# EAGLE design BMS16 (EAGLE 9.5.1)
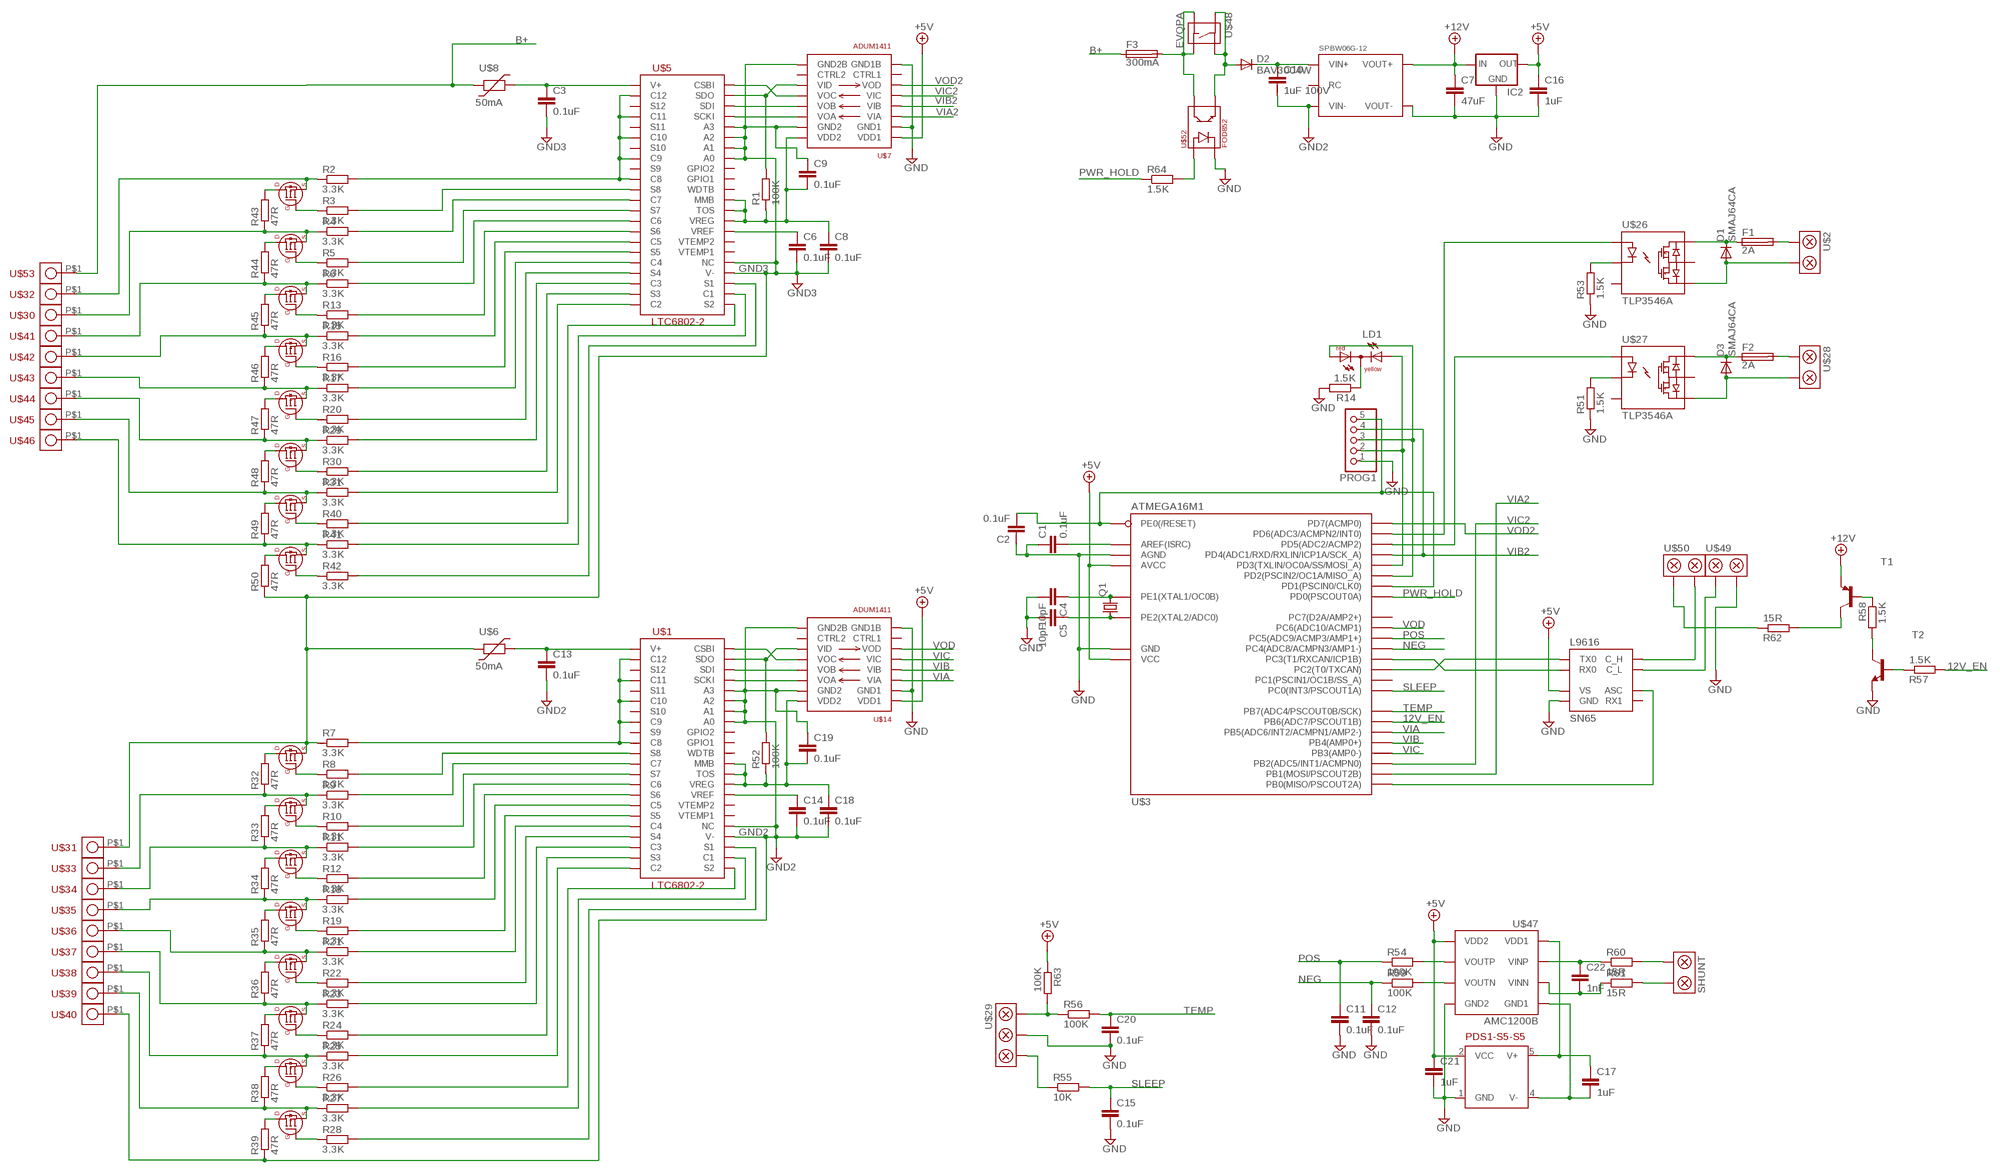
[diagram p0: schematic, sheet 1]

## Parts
C1  0.1uF  C-EUC1206  [C1206]
C2  0.1uF  C-EUC1206  [C1206]
C3  0.1uF  C-EUC1206  [C1206]
C4  10pF  C-EUC0805  [C0805]
C5  10pF  C-EUC0805  [C0805]
C6  0.1uF  C-EUC1206  [C1206]
C7  47uF  C-EUC1206  [C1206]
C8  0.1uF  C-EUC1206  [C1206]
C9  0.1uF  C-EUC1206  [C1206]
C10  1uF 100V  C-EUC1206  [C1206]
C11  0.1uF  C-EUC1206  [C1206]
C12  0.1uF  C-EUC1206  [C1206]
C13  0.1uF  C-EUC1206  [C1206]
C14  0.1uF  C-EUC1206  [C1206]
C15  0.1uF  C-EUC1206  [C1206]
C16  1uF  C-EUC1206  [C1206]
C17  1uF  C-EUC1206  [C1206]
C18  0.1uF  C-EUC1206  [C1206]
C19  0.1uF  C-EUC1206  [C1206]
C20  0.1uF  C-EUC1206  [C1206]
C21  1uF  C-EUC1206  [C1206]
C22  1nF  C-EUC1206  [C1206]
D1  SMAJ64CA  DIODE-DO214AC  [DO214AC]
D2  BAV3004W  DIODE-SOD123  [SOD123]
D3  SMAJ64CA  DIODE-DO214AC  [DO214AC]
F1  2A  TE5  [TE5]
F2  2A  TE5  [TE5]
F3  300mA  TE5  [TE5]
IC2  78LXXSOT89  [SOT89R]
LD1  DUOLED-RY-C  [DUOLED-C-5MM]
PDS1-S5-S5  PDS2  [PDS2]
PROG1  PINHD-1X5  [1X05]
Q1  CRYSTALCTS406  [CTS406]
R1  100K  R-EU_R1206  [R1206]
R2  3.3K  R-EU_R1206  [R1206]
R3  3.3K  R-EU_R1206  [R1206]
R4  3.3K  R-EU_R1206  [R1206]
R5  3.3K  R-EU_R1206  [R1206]
R6  3.3K  R-EU_R1206  [R1206]
R7  3.3K  R-EU_R1206  [R1206]
R8  3.3K  R-EU_R1206  [R1206]
R9  3.3K  R-EU_R1206  [R1206]
R10  3.3K  R-EU_R1206  [R1206]
R11  3.3K  R-EU_R1206  [R1206]
R12  3.3K  R-EU_R1206  [R1206]
R13  3.3K  R-EU_R1206  [R1206]
R14  1.5K  R-EU_R1206  [R1206]
R15  3.3K  R-EU_R1206  [R1206]
R16  3.3K  R-EU_R1206  [R1206]
R17  3.3K  R-EU_R1206  [R1206]
R18  3.3K  R-EU_R1206  [R1206]
R19  3.3K  R-EU_R1206  [R1206]
R20  3.3K  R-EU_R1206  [R1206]
R21  3.3K  R-EU_R1206  [R1206]
R22  3.3K  R-EU_R1206  [R1206]
R23  3.3K  R-EU_R1206  [R1206]
R24  3.3K  R-EU_R1206  [R1206]
R25  3.3K  R-EU_R1206  [R1206]
R26  3.3K  R-EU_R1206  [R1206]
R27  3.3K  R-EU_R1206  [R1206]
R28  3.3K  R-EU_R1206  [R1206]
R29  3.3K  R-EU_R1206  [R1206]
R30  3.3K  R-EU_R1206  [R1206]
R31  3.3K  R-EU_R1206  [R1206]
R32  47R  R-EU_R2512  [R2512]
R33  47R  R-EU_R2512  [R2512]
R34  47R  R-EU_R2512  [R2512]
R35  47R  R-EU_R2512  [R2512]
R36  47R  R-EU_R2512  [R2512]
R37  47R  R-EU_R2512  [R2512]
R38  47R  R-EU_R2512  [R2512]
R39  47R  R-EU_R2512  [R2512]
R40  3.3K  R-EU_R1206  [R1206]
R41  3.3K  R-EU_R1206  [R1206]
R42  3.3K  R-EU_R1206  [R1206]
R43  47R  R-EU_R2512  [R2512]
R44  47R  R-EU_R2512  [R2512]
R45  47R  R-EU_R2512  [R2512]
R46  47R  R-EU_R2512  [R2512]
R47  47R  R-EU_R2512  [R2512]
R48  47R  R-EU_R2512  [R2512]
R49  47R  R-EU_R2512  [R2512]
R50  47R  R-EU_R2512  [R2512]
R51  1.5K  R-EU_R1206  [R1206]
R52  100K  R-EU_R1206  [R1206]
R53  1.5K  R-EU_R1206  [R1206]
R54  100K  R-EU_R1206  [R1206]
R55  10K  R-EU_R1206  [R1206]
R56  100K  R-EU_R1206  [R1206]
R57  1.5K  R-EU_R1206  [R1206]
R58  1.5K  R-EU_R1206  [R1206]
R59  100K  R-EU_R1206  [R1206]
R60  15R  R-EU_R1206  [R1206]
R61  15R  R-EU_R1206  [R1206]
R62  15R  R-EU_R1206  [R1206]
R63  100K  R-EU_R1206  [R1206]
R64  1.5K  R-EU_R1206  [R1206]
SHUNT  SCREWTERM_2WAY5MM  [SCREWTERM_5MM_2WAY]
SN65  L9616  [SOIC8]
SPBW06G-12  SPBW06  [SPBW06]
T1  MMBT540LT1-PNP-SOT23-BEC  [SOT23-BEC]
T2  MMBT4401LT1-NPN-SOT23-BEC  [SOT23-BEC]
U$1  LTC6802-2  [SSOP-44]
U$2  SCREWTERM_2WAY5MM  [SCREWTERM_5MM_2WAY]
U$3  ATMEGA16M1  [TQFP32]
U$5  LTC6802-2  [SSOP-44]
U$6  50mA  1206_POLYSWITCH  [1206]
U$7  ADUM1411  [SOIC16W]
U$8  50mA  1206_POLYSWITCH  [1206]
U$9  SI2351DS  [SOT23]
U$10  SI2351DS  [SOT23]
U$11  SI2351DS  [SOT23]
U$12  SI2351DS  [SOT23]
U$13  SI2351DS  [SOT23]
U$14  ADUM1411  [SOIC16W]
U$15  SI2351DS  [SOT23]
U$16  SI2351DS  [SOT23]
U$17  SI2351DS  [SOT23]
U$18  SI2351DS  [SOT23]
U$19  SI2351DS  [SOT23]
U$20  SI2351DS  [SOT23]
U$21  SI2351DS  [SOT23]
U$22  SI2351DS  [SOT23]
U$23  SI2351DS  [SOT23]
U$24  SI2351DS  [SOT23]
U$25  SI2351DS  [SOT23]
U$26  TLP3546A  AQV252GA  [SMD6]
U$27  TLP3546A  AQV252GA  [SMD6]
U$28  SCREWTERM_2WAY5MM  [SCREWTERM_5MM_2WAY]
U$29  SCREWTERM_3WAY5MM  [SCREWTERM_5MM_3WAY]
U$30  PHOENIX_508_SCREW_PLUG_1  [PHOENIX_508_SCREW_PLUG_1]
U$31  PHOENIX_508_SCREW_PLUG_1  [PHOENIX_508_SCREW_PLUG_1]
U$32  PHOENIX_508_SCREW_PLUG_1  [PHOENIX_508_SCREW_PLUG_1]
U$33  PHOENIX_508_SCREW_PLUG_1  [PHOENIX_508_SCREW_PLUG_1]
U$34  PHOENIX_508_SCREW_PLUG_1  [PHOENIX_508_SCREW_PLUG_1]
U$35  PHOENIX_508_SCREW_PLUG_1  [PHOENIX_508_SCREW_PLUG_1]
U$36  PHOENIX_508_SCREW_PLUG_1  [PHOENIX_508_SCREW_PLUG_1]
U$37  PHOENIX_508_SCREW_PLUG_1  [PHOENIX_508_SCREW_PLUG_1]
U$38  PHOENIX_508_SCREW_PLUG_1  [PHOENIX_508_SCREW_PLUG_1]
U$39  PHOENIX_508_SCREW_PLUG_1  [PHOENIX_508_SCREW_PLUG_1]
U$40  PHOENIX_508_SCREW_PLUG_1  [PHOENIX_508_SCREW_PLUG_1]
U$41  PHOENIX_508_SCREW_PLUG_1  [PHOENIX_508_SCREW_PLUG_1]
U$42  PHOENIX_508_SCREW_PLUG_1  [PHOENIX_508_SCREW_PLUG_1]
U$43  PHOENIX_508_SCREW_PLUG_1  [PHOENIX_508_SCREW_PLUG_1]
U$44  PHOENIX_508_SCREW_PLUG_1  [PHOENIX_508_SCREW_PLUG_1]
U$45  PHOENIX_508_SCREW_PLUG_1  [PHOENIX_508_SCREW_PLUG_1]
U$46  PHOENIX_508_SCREW_PLUG_1  [PHOENIX_508_SCREW_PLUG_1]
U$47  AMC1200B  AMC1200  [SOIC8W]
U$48  EVQPA  [EVQPA]
U$49  SCREWTERM_2WAY5MM  [SCREWTERM_5MM_2WAY]
U$50  SCREWTERM_2WAY5MM  [SCREWTERM_5MM_2WAY]
U$52  FOD852  [SMD4]
U$53  PHOENIX_508_SCREW_PLUG_1  [PHOENIX_508_SCREW_PLUG_1]

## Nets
12V_EN: R57.2 U$3.27(PB6(ADC7/PSCOUT1B))
+5V: C16.1 C21.1 IC2.2(OUT) PDS1-S5-S5.2(VCC) R63.1 SN65.P$3(VS) U$3.4(VCC) U$3.19(AVCC) U$7.1(VDD1) U$14.1(VDD1) U$47.8(VDD2)
+12V: C7.1 IC2.1(IN) SPBW06G-12.6(VOUT+) T1.E
B+: F3.1 U$8.P$1 U$53.P$1
FD: F3.2 U$48.A U$48.A2 U$52.P$4(COL)
FDS: C3.1 U$5.1(V+) U$8.P$2
FS: R2.1 U$18.P$2(S) U$32.P$1
GND: C1.1 C2.1 C4.2 C5.2 C7.2 C11.2 C12.2 C15.2 C16.2 C20.2 C21.2 IC2.4(GND) PDS1-S5-S5.1(GND) PROG1.1 R14.2 R51.1 R53.1 SN65.P$2(GND) SPBW06G-12.7(VOUT-) T2.E U$3.5(GND) U$3.20(AGND) U$7.2(GND1) U$7.8(GND1B) U$14.2(GND1) U$14.8(GND1B) U$29.P$2 U$47.5(GND2) U$49.P$1 U$52.P$2(CAT)
GND2: C10.2 C13.2 C14.2 C18.2 C19.1 R39.1 SPBW06G-12.1(VIN-) U$1.26(V-) U$1.27(NC) U$1.37(A0) U$1.38(A1) U$1.39(A2) U$1.40(A3) U$14.9(GND2B) U$14.15(GND2) U$40.P$1
GND3: C3.2 C6.2 C8.2 C9.1 R7.1 R50.1 U$5.26(V-) U$5.27(NC) U$5.37(A0) U$5.38(A1) U$5.39(A2) U$5.40(A3) U$6.P$1 U$7.9(GND2B) U$7.15(GND2) U$9.P$2(S) U$31.P$1
N$1: D1.C F1.1 U$26.6
N$2: R7.2 U$1.2(C12) U$1.4(C11) U$1.6(C10) U$1.8(C9) U$1.10(C8)
N$3: C22.1 R60.1 U$47.2(VINP)
N$4: U$5.42(SDI) U$7.13(VOB)
N$5: U$5.41(SCKI) U$7.14(VOA)
N$6: R1.2 U$5.43(SDO) U$7.11(VID)
N$7: U$1.42(SDI) U$14.13(VOB)
N$8: U$5.44(CSBI) U$7.12(VOC)
N$9: C8.1 C9.2 R1.1 U$5.31(VREG) U$5.32(TOS) U$5.33(MMB) U$7.16(VDD2)
N$10: R26.2 U$1.23(S2)
N$11: U$1.41(SCKI) U$14.14(VOA)
N$12: R27.2 U$1.24(C1)
N$13: R28.2 U$1.25(S1)
N$14: C6.1 U$5.30(VREF)
N$15: R52.2 U$1.43(SDO) U$14.11(VID)
N$16: U$1.44(CSBI) U$14.12(VOC)
N$17: R40.2 U$5.23(S2)
N$18: R41.2 U$5.24(C1)
N$19: C2.2 PROG1.5 U$3.31(PE0(/RESET)) U$3.32(PD1(PSCIN0/CLK0))
N$20: F1.2 U$2.P$2
N$21: R42.2 U$5.25(S1)
N$22: R4.2 U$5.12(C7)
N$23: R9.2 U$1.12(C7)
N$24: R11.2 U$1.14(C6)
N$25: C18.1 C19.2 R52.1 U$1.31(VREG) U$1.32(TOS) U$1.33(MMB) U$14.16(VDD2)
N$26: R18.2 U$1.16(C5)
N$27: R21.2 U$1.18(C4)
N$28: R23.2 U$1.20(C3)
N$29: R25.2 U$1.22(C2)
N$30: R6.2 U$5.14(C6)
N$31: R15.2 U$5.16(C5)
N$32: LD1.AX(AY) PROG1.2 U$3.2(PD3(TXLIN/OC0A/SS/MOSI_A))
N$33: LD1.AR PROG1.3 U$3.1(PD2(PSCIN2/OC1A/MISO_A))
N$34: F2.2 U$28.P$2
N$35: C1.2 U$3.21(AREF(ISRC))
N$36: SN65.P$4(RX0) U$3.7(PC3(T1/RXCAN/ICP1B))
N$37: SN65.P$1(TX0) U$3.6(PC2(T0/TXCAN))
N$38: SN65.P$7(C_H) U$50.P$1
N$39: SN65.P$6(C_L) U$49.P$2
N$40: C22.2 R61.1 U$47.3(VINN)
N$41: R55.1 U$29.P$1
N$42: C10.1 D2.C SPBW06G-12.2(VIN+)
N$43: D2.A U$48.B U$48.B2 U$52.P$3(EM)
N$44: R62.1 U$50.P$2
N$45: LD1.C R14.1
N$46: R17.2 U$5.18(C4)
N$47: SN65.P$8(ASC) U$3.8(PB0(MISO/PSCOUT2A))
N$48: C4.1 Q1.3 U$3.10(PE1(XTAL1/OC0B))
N$49: C5.1 Q1.1 U$3.11(PE2(XTAL2/ADC0))
N$50: R29.2 U$5.20(C3)
N$51: R31.2 U$5.22(C2)
N$52: R54.2 U$47.7(VOUTP)
N$53: D1.A U$2.P$1 U$26.4
N$54: R3.1 U$18.P$1(G)
N$55: R5.1 U$19.P$1(G)
N$56: R13.1 U$20.P$1(G)
N$57: R8.1 U$9.P$1(G)
N$58: R10.1 U$10.P$1(G)
N$59: R12.1 U$11.P$1(G)
N$60: R28.1 U$17.P$1(G)
N$61: R19.1 U$12.P$1(G)
N$62: R22.1 U$13.P$1(G)
N$63: R24.1 U$15.P$1(G)
N$64: R26.1 U$16.P$1(G)
N$65: R27.1 R38.1 U$17.P$2(S) U$39.P$1
N$66: C14.1 U$1.30(VREF)
N$67: R42.1 U$25.P$1(G)
N$68: R16.1 U$21.P$1(G)
N$69: R25.1 R37.1 U$16.P$2(S) U$38.P$1
N$70: R23.1 R36.1 U$15.P$2(S) U$37.P$1
N$71: R38.2 U$16.P$3(D)
N$72: R39.2 U$17.P$3(D)
N$73: R37.2 U$15.P$3(D)
N$74: R21.1 R35.1 U$13.P$2(S) U$36.P$1
N$75: R36.2 U$13.P$3(D)
N$76: R18.1 R34.1 U$12.P$2(S) U$35.P$1
N$77: R35.2 U$12.P$3(D)
N$78: R11.1 R33.1 U$11.P$2(S) U$34.P$1
N$79: R9.1 R32.1 U$10.P$2(S) U$33.P$1
N$80: R33.2 U$10.P$3(D)
N$81: R34.2 U$11.P$3(D)
N$82: R32.2 U$9.P$3(D)
N$83: R24.2 U$1.21(S3)
N$84: R22.2 U$1.19(S4)
N$85: R20.1 U$22.P$1(G)
N$86: R30.1 U$23.P$1(G)
N$87: R40.1 U$24.P$1(G)
N$88: R41.1 R49.1 U$25.P$2(S) U$46.P$1
N$89: R8.2 U$1.11(S8)
N$90: R10.2 U$1.13(S7)
N$91: R12.2 U$1.15(S6)
N$92: R31.1 R48.1 U$24.P$2(S) U$45.P$1
N$93: R19.2 U$1.17(S5)
N$94: R29.1 R47.1 U$23.P$2(S) U$44.P$1
N$95: R49.2 U$24.P$3(D)
N$96: R50.2 U$25.P$3(D)
N$97: R48.2 U$23.P$3(D)
N$98: R17.1 R46.1 U$22.P$2(S) U$43.P$1
N$99: R47.2 U$22.P$3(D)
N$100: R15.1 R45.1 U$21.P$2(S) U$42.P$1
N$101: R46.2 U$21.P$3(D)
N$102: R6.1 R44.1 U$20.P$2(S) U$41.P$1
N$103: R4.1 R43.1 U$19.P$2(S) U$30.P$1
N$104: R44.2 U$19.P$3(D)
N$105: R45.2 U$20.P$3(D)
N$106: R43.2 U$18.P$3(D)
N$107: R3.2 U$5.11(S8)
N$108: R5.2 U$5.13(S7)
N$109: R13.2 U$5.15(S6)
N$110: R16.2 U$5.17(S5)
N$111: R20.2 U$5.19(S4)
N$112: R30.2 U$5.21(S3)
N$113: R2.2 U$5.2(C12) U$5.4(C11) U$5.6(C10) U$5.8(C9) U$5.10(C8)
N$114: R56.1 R63.2 U$29.P$3
N$115: D3.C F2.1 U$27.6
N$116: C17.1 PDS1-S5-S5.5(V+) U$47.1(VDD1)
N$117: D3.A U$27.4 U$28.P$1
N$118: U$3.14(PD6(ADC3/ACMPN2/INT0)) U$26.1
N$119: U$3.13(PD5(ADC2/ACMP2)) U$27.1
N$120: R53.2 U$26.2
N$121: R51.2 U$27.2
N$122: R57.1 T2.B
N$123: R58.2 T2.C
N$124: C17.2 PDS1-S5-S5.4(V-) U$47.4(GND1)
N$125: R58.1 T1.B
N$126: R62.2 T1.C
N$127: R59.2 U$47.6(VOUTN)
N$128: R64.2 U$52.P$1(AN)
N$129: R61.2 SHUNT.P$2
N$130: R60.2 SHUNT.P$1
NEG: C12.1 R59.1 U$3.17(PC4(ADC8/ACMPN3/AMP1-))
POS: C11.1 R54.1 U$3.18(PC5(ADC9/ACMP3/AMP1+))
PWR_HOLD: R64.1 U$3.29(PD0(PSCOUT0A))
SLEEP: C15.1 R55.2 U$3.30(PC0(INT3/PSCOUT1A))
TEMP: C20.1 R56.2 U$3.28(PB7(ADC4/PSCOUT0B/SCK))
V+: C13.1 U$1.1(V+) U$6.P$2
VIA: U$3.26(PB5(ADC6/INT2/ACMPN1/AMP2-)) U$14.3(VIA)
VIA2: U$3.9(PB1(MOSI/PSCOUT2B)) U$7.3(VIA)
VIB: U$3.24(PB4(AMP0+)) U$14.4(VIB)
VIB2: PROG1.4 U$3.12(PD4(ADC1/RXD/RXLIN/ICP1A/SCK_A)) U$7.4(VIB)
VIC: U$3.23(PB3(AMP0-)) U$14.5(VIC)
VIC2: U$3.16(PB2(ADC5/INT1/ACMPN0)) U$7.5(VIC)
VOD: U$3.22(PC6(ADC10/ACMP1)) U$14.6(VOD)
VOD2: U$3.15(PD7(ACMP0)) U$7.6(VOD)
Unconnected: SN65.P$5(RX1) SPBW06G-12.3(RC) U$1.3(S12) U$1.5(S11) U$1.7(S10) U$1.9(S9) U$1.28(VTEMP1) U$1.29(VTEMP2) U$1.34(WDTB) U$1.35(GPIO1) U$1.36(GPIO2) U$3.3(PC1(PSCIN1/OC1B/SS_A)) U$3.25(PC7(D2A/AMP2+)) U$5.3(S12) U$5.5(S11) U$5.7(S10) U$5.9(S9) U$5.28(VTEMP1) U$5.29(VTEMP2) U$5.34(WDTB) U$5.35(GPIO1) U$5.36(GPIO2) U$7.7(CTRL1) U$7.10(CTRL2) U$14.7(CTRL1) U$14.10(CTRL2) U$26.3 U$26.5 U$27.3 U$27.5

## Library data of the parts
C1-C22 = resistor:C-EU: CAPACITOR, European symbol
D1-D3 = diode:DIODE-: DIODE
F1-F3 = fuse:TE5: FUSE
IC2 = v-reg:78LXX: VOLTAGE REGULATOR
LD1 = led:DUOLED-RY-C: DUO LED 2 colors (red/yellow), 5 mm, round, common Cathode www.ligitek.com or other producers.
PDS1-S5-S5 = Ians parts:PDS2
PROG1 = pinhead:PINHD-1X5: PIN HEADER
Q1 = crystal:CRYSTAL: CRYSTAL
R1-R64 = resistor:R-EU_: RESISTOR, European symbol
SHUNT U$2 U$28 U$49 U$50 = Ians parts:SCREWTERM_2WAY
SN65 = Ians parts:L9616
SPBW06G-12 = Ians parts:SPBW06
T1 = transistor:*-PNP-: PNP Transistror
T2 = transistor:*-NPN-: NPN Transistror BF959 corrected 2008.03.06
U$1 U$5 = Ians parts:LTC6802-2
U$3 = Ians parts:ATMEGA16M1
U$6 U$8 = Ians parts:1206_POLYSWITCH
U$7 U$14 = Ians parts:ADUM1411
U$9-U$13 U$15-U$25 = Ians parts:SI2351DS
U$26 U$27 = Ians parts:AQV252GA
U$29 = Ians parts:SCREWTERM_3WAY
U$30-U$46 U$53 = Ians parts:PHOENIX_508_SCREW_PLUG_1
U$47 = Ians parts:AMC1200
U$48 = Ians parts:EVQPA
U$52 = Ians parts:FOD852

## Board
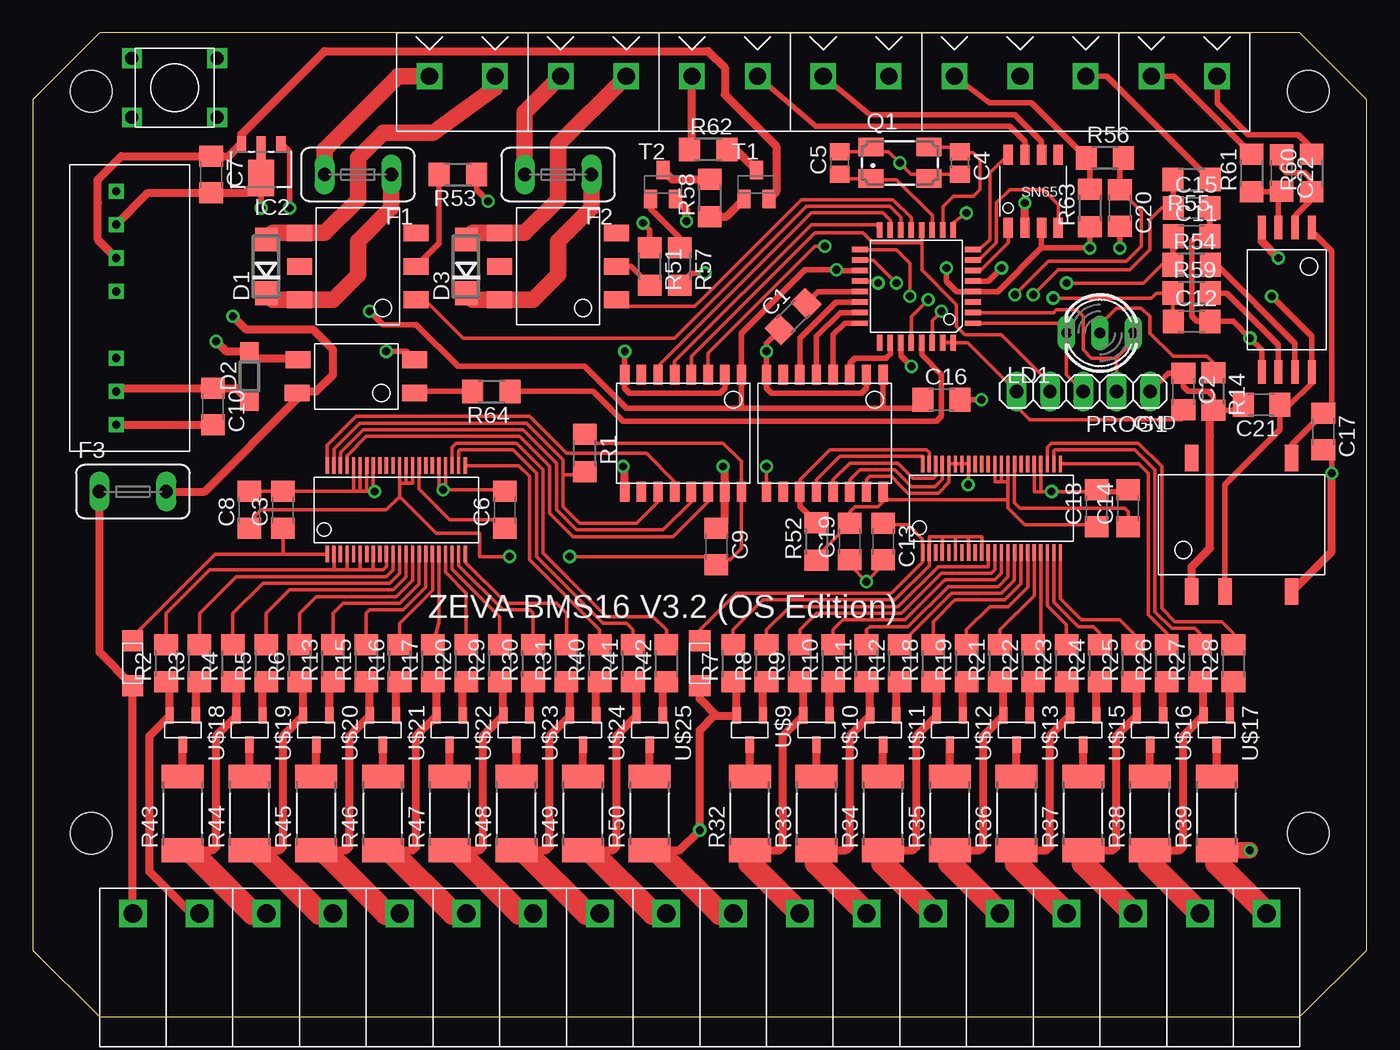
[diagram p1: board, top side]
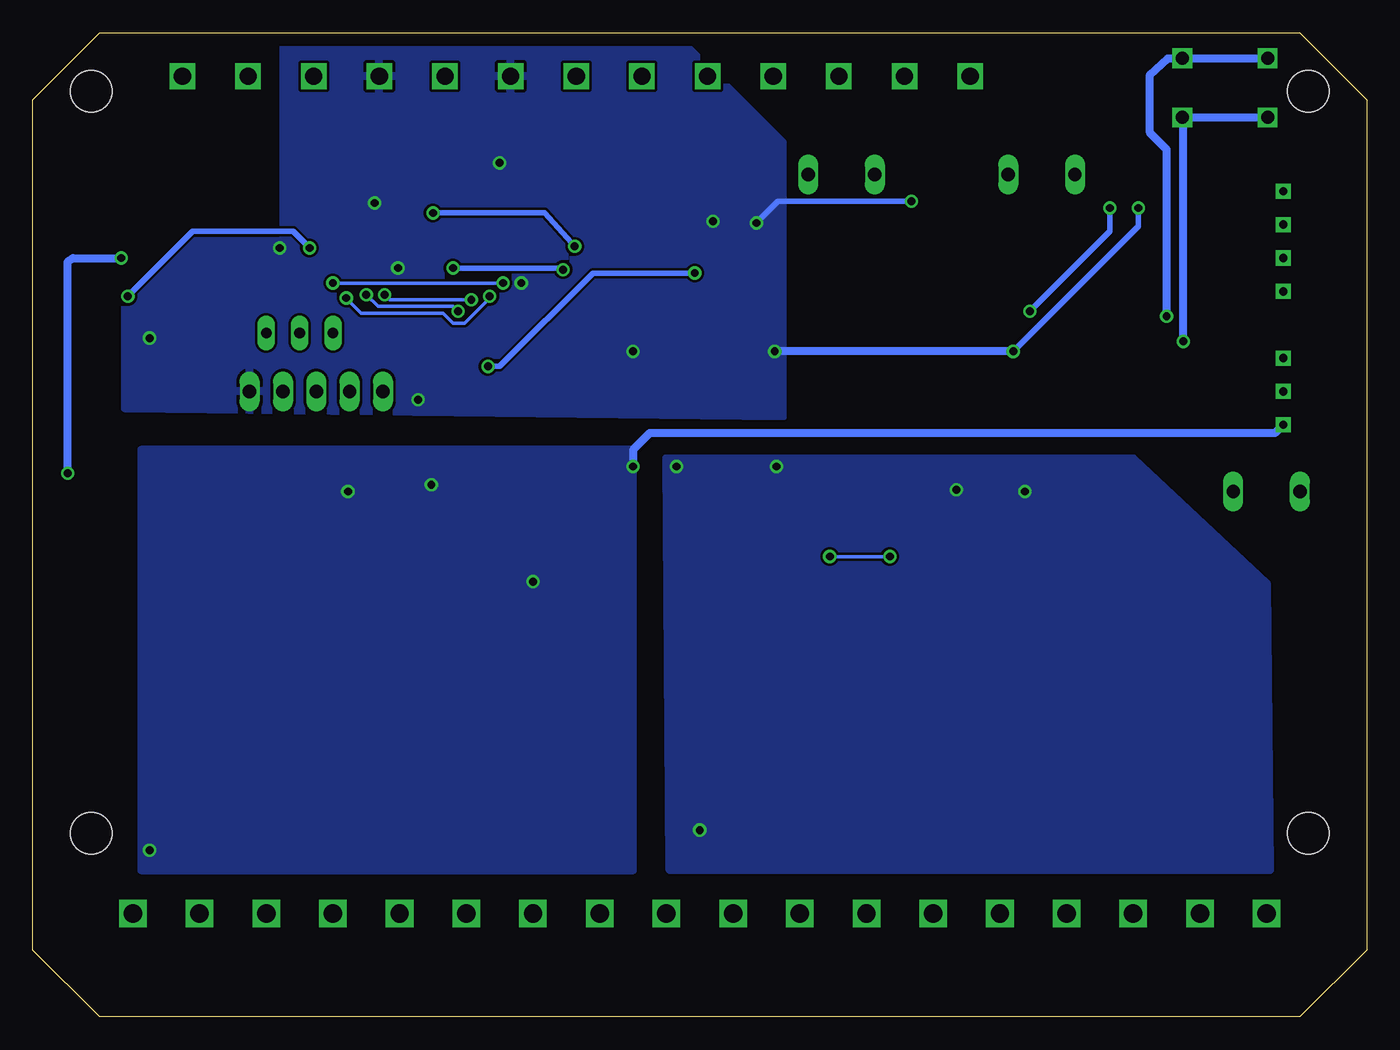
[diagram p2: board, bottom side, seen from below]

Size 101.6 x 74.93 mm. Coordinates in mm from the lower left corner, seen from the top.
Outline: 0,5.08 5.08,0 96.52,0 101.6,5.08 101.6,69.85 96.52,74.93 5.08,74.93 0,69.85 0,5.08
Copper layers (1*16): Top 0.035mm / dielectric 1.5mm / Bottom 0.035mm
Design rules "default *": minimum track width 10mil, minimum drill 10mil, track to track 8mil, track to pad 8mil, pad to pad 8mil, via to via 8mil, smd to smd 8mil, copper to edge 40mil, drill to drill 8mil, minimum pad ring 10mil, minimum via ring 8mil, stop-mask expansion 4mil, vias tented up to drill 0mil, thermal gap 10mil
Holes 3.17 mm at 97.16,13.97 97.16,70.48 4.45,70.48 4.45,13.97

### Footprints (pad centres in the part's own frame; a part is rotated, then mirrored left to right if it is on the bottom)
C1206 = smd 1.6 x 1.8: 1 -1.4,0; 2 1.4,0
C0805 = smd 1.3 x 1.5: 1 -0.85,0; 2 0.85,0
DO214AC = smd 1.8 x 1.7: A 2.05,0; C -2.05,0
SOD123 = smd 1.4 x 1.4: A 1.9,0; C -1.9,0
TE5 = drill 1.016 long: 1 -2.54,0; 2 2.54,0
SOT89R = smd 0.7 x 1.1: 1 1.5,-1.75; 2 -1.5,-1.75 | smd 0.7 x 1.8: 3 0,-1.4 | smd 2 x 2.8: 4 0,0.9
DUOLED-C-5MM = drill 0.813 long: AR 2.54,0; AX -2.54,0; C 0,0
PDS2 = smd 1.016 x 2.032: 1 -3.81,-5.08; 2 -1.27,-5.08; 4 3.81,-5.08; 5 3.81,5.08; 8 -3.81,5.08
1X05 = drill 1.016 long: 1 -5.08,0; 2 -2.54,0; 3 0,0; 4 2.54,0; 5 5.08,0
CTS406 = smd 1.9 x 1.4: 1 -2.2,-1.2; 2 2.2,-1.2; 3 2.2,1.2; 4 -2.2,1.2
R1206 = smd 1.6 x 1.803: 1 -1.422,0; 2 1.422,0
R2512 = smd 1.8 x 3.2: 1 -2.8,0; 2 2.8,0
SCREWTERM_5MM_2WAY = drill 1.3 square: P$1 -2.5,0; P$2 2.5,0
SOIC8 = smd 1.524 x 0.711: P$1 -2.794,1.905; P$2 -2.794,0.635; P$3 -2.794,-0.635; P$4 -2.794,-1.905; P$5 2.794,-1.905; P$6 2.794,-0.635; P$7 2.794,0.635; P$8 2.794,1.905
SPBW06 = drill 0.635 square: 1 0,8.89; 2 0,6.35; 3 0,3.81; 5 0,-1.27; 6 0,-3.81; 7 0,-6.35; 8 0,-8.89
SOT23-BEC = smd 1 x 1.4: B -0.95,-1.1; C 0,1.1; E 0.95,-1.1
SSOP-44 = smd 1.25 x 0.25: 1 -3.375,5.25; 2 -3.375,4.75; 3 -3.375,4.25; 4 -3.375,3.75; 5 -3.375,3.25; 6 -3.375,2.75; 7 -3.375,2.25; 8 -3.375,1.75; 9 -3.375,1.25; 10 -3.375,0.75; 11 -3.375,0.25; 12 -3.375,-0.25; 13 -3.375,-0.75; 14 -3.375,-1.25; 15 -3.375,-1.75; 16 -3.375,-2.25; 17 -3.375,-2.75; 18 -3.375,-3.25; 19 -3.375,-3.75; 20 -3.375,-4.25; 21 -3.375,-4.75; 22 -3.375,-5.25; 23 3.375,-5.25; 24 3.375,-4.75; 25 3.375,-4.25; 26 3.375,-3.75; 27 3.375,-3.25; 28 3.375,-2.75; 29 3.375,-2.25; 30 3.375,-1.75; 31 3.375,-1.25; 32 3.375,-0.75; 33 3.375,-0.25; 34 3.375,0.25; 35 3.375,0.75; 36 3.375,1.25; 37 3.375,1.75; 38 3.375,2.25; 39 3.375,2.75; 40 3.375,3.25; 41 3.375,3.75; 42 3.375,4.25; 43 3.375,4.75; 44 3.375,5.25
TQFP32 = smd 1.2 x 0.4: 1 -4.3,2.8; 2 -4.3,2; 3 -4.3,1.2; 4 -4.3,0.4; 5 -4.3,-0.4; 6 -4.3,-1.2; 7 -4.3,-2; 8 -4.3,-2.8; 17 4.3,-2.8; 18 4.3,-2; 19 4.3,-1.2; 20 4.3,-0.4; 21 4.3,0.4; 22 4.3,1.2; 23 4.3,2; 24 4.3,2.8 | smd 0.4 x 1.2: 9 -2.8,-4.3; 10 -2,-4.3; 11 -1.2,-4.3; 12 -0.4,-4.3; 13 0.4,-4.3; 14 1.2,-4.3; 15 2,-4.3; 16 2.8,-4.3; 25 2.8,4.3; 26 2,4.3; 27 1.2,4.3; 28 0.4,4.3; 29 -0.4,4.3; 30 -1.2,4.3; 31 -2,4.3; 32 -2.8,4.3
1206 = smd 1.6 x 1.6: P$1 -1.7,0; P$2 1.7,0
SOIC16W = smd 1.524 x 0.711: 1 -4.445,4.445; 2 -4.445,3.175; 3 -4.445,1.905; 4 -4.445,0.635; 5 -4.445,-0.635; 6 -4.445,-1.905; 7 -4.445,-3.175; 8 -4.445,-4.445; 9 4.445,-4.445; 10 4.445,-3.175; 11 4.445,-1.905; 12 4.445,-0.635; 13 4.445,0.635; 14 4.445,1.905; 15 4.445,3.175; 16 4.445,4.445
SOT23 = smd 1.27 x 0.635: P$1 -1.1,1; P$2 -1.1,-1; P$3 1.1,0
SMD6 = smd 1.905 x 1.27: 1 -4.445,2.54; 2 -4.445,0; 3 -4.445,-2.54; 4 4.445,-2.54; 5 4.445,0; 6 4.445,2.54
SCREWTERM_5MM_3WAY = drill 1.3 square: P$1 -5,0; P$2 0,0; P$3 5,0
PHOENIX_508_SCREW_PLUG_1 = drill 1.4 square: P$1 0,0
SOIC8W = smd 1.8 x 0.6: 1 -5.5,1.905; 2 -5.5,0.635; 3 -5.5,-0.635; 4 -5.5,-1.905; 5 5.5,-1.905; 6 5.5,-0.635; 7 5.5,0.635; 8 5.5,1.905
EVQPA = drill 1 square: A -2.25,3.25; A2 -2.25,-3.25; B 2.25,3.25; B2 2.25,-3.25
SMD4 = smd 1.905 x 1.27: P$1 -4.445,1.27; P$2 -4.445,-1.27; P$3 4.445,-1.27; P$4 4.5,1.27

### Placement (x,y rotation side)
C1  57.91,53.34 45 top
C2  87.63,47.62 270 top
C3  19.05,38.61 90 top
C4  70.61,65.02 270 top
C5  61.47,65.02 90 top
C6  35.94,38.61 90 top
C7  13.59,64.14 270 top
C8  16.51,38.61 90 top
C9  52.07,35.81 270 top
C10  13.72,46.48 270 top
C11  88.27,59.44 0 top
C12  88.27,52.96 0 top
C13  64.77,36.2 270 top
C14  83.44,38.73 90 top
C15  88.27,61.59 0 top
C16  69.22,46.99 0 top
C17  98.3,44.58 270 top
C18  81.03,38.73 90 top
C19  62.23,36.2 90 top
C20  82.8,61.59 270 top
C21  93.6,46.61 180 top
C22  95.12,64.26 270 top
D1  17.78,57.15 90 top
D2  16.51,48.77 90 top
D3  33.02,57.15 90 top
F1  24.77,64.14 180 top
F2  40.01,64.14 180 top
F3  7.62,40.01 0 top
IC2  17.4,64.77 180 top
LD1  81.28,52.07 180 top
PDS1-S5-S5  92.08,37.47 0 top
PROG1  80.01,47.62 180 top
Q1  66.04,65.02 0 top
R1  42.04,42.93 270 top
R2  10.16,26.92 90 top
R3  12.7,26.92 90 top
R4  15.24,26.92 90 top
R5  17.78,26.92 90 top
R6  20.32,26.92 90 top
R7  53.34,26.92 90 top
R8  55.88,26.92 90 top
R9  58.42,26.92 90 top
R10  60.96,26.92 90 top
R11  63.5,26.92 90 top
R12  66.04,26.92 90 top
R13  22.86,26.92 90 top
R14  89.92,47.62 270 top
R15  25.4,26.92 90 top
R16  27.94,26.92 90 top
R17  30.48,26.92 90 top
R18  68.58,26.92 90 top
R19  71.12,26.92 90 top
R20  33.02,26.92 90 top
R21  73.66,26.92 90 top
R22  76.2,26.92 90 top
R23  78.74,26.92 90 top
R24  81.28,26.92 90 top
R25  83.82,26.92 90 top
R26  86.36,26.92 90 top
R27  88.9,26.92 90 top
R28  91.44,26.92 90 top
R29  35.56,26.92 90 top
R30  38.1,26.92 90 top
R31  40.64,26.92 90 top
R32  54.61,15.49 90 top
R33  59.69,15.49 90 top
R34  64.77,15.49 90 top
R35  69.85,15.49 90 top
R36  74.93,15.49 90 top
R37  80.01,15.49 90 top
R38  85.09,15.49 90 top
R39  90.17,15.49 90 top
R40  43.18,26.92 90 top
R41  45.72,26.92 90 top
R42  48.26,26.92 90 top
R43  11.43,15.49 90 top
R44  16.51,15.49 90 top
R45  21.59,15.49 90 top
R46  26.67,15.49 90 top
R47  31.75,15.49 90 top
R48  36.83,15.49 90 top
R49  41.91,15.49 90 top
R50  46.99,15.49 90 top
R51  46.99,57.15 270 top
R52  59.69,36.2 90 top
R53  32.38,64.14 180 top
R54  88.27,57.28 0 top
R55  88.27,63.75 180 top
R56  81.66,65.41 0 top
R57  49.28,57.15 270 top
R58  51.56,62.36 90 top
R59  88.27,55.12 0 top
R60  97.41,64.26 90 top
R61  92.84,64.26 90 top
R62  51.44,66.04 0 top
R63  80.52,61.59 90 top
R64  34.92,47.62 180 top
SHUNT  87.7,71.63 180 top
SN65  76.2,62.87 90 top
SPBW06G-12  6.35,53.98 180 top
T1  55.12,63.37 0 top
T2  48.01,63.37 0 top
U$1  73.03,38.73 90 top
U$2  32.7,71.63 180 top
U$3  67.31,55.63 180 top
U$5  27.69,38.61 90 top
U$6  50.8,26.92 90 top
U$7  49.53,44.45 270 top
U$8  7.62,26.92 90 top
U$9  54.61,21.84 270 top
U$10  59.69,21.84 270 top
U$11  64.77,21.84 270 top
U$12  69.85,21.84 270 top
U$13  74.93,21.84 270 top
U$14  60.33,44.45 270 top
U$15  80.01,21.84 270 top
U$16  85.09,21.84 270 top
U$17  90.17,21.84 270 top
U$18  11.43,21.84 270 top
U$19  16.51,21.84 270 top
U$20  21.59,21.84 270 top
U$21  26.67,21.84 270 top
U$22  31.75,21.84 270 top
U$23  36.83,21.84 270 top
U$24  41.91,21.84 270 top
U$25  46.99,21.84 270 top
U$26  24.77,57.15 180 top
U$27  40.01,57.15 180 top
U$28  42.7,71.63 180 top
U$29  75.2,71.63 180 top
U$30  17.78,7.87 0 top
U$31  53.34,7.87 0 top
U$32  12.7,7.87 0 top
U$33  58.42,7.87 0 top
U$34  63.5,7.87 0 top
U$35  68.58,7.87 0 top
U$36  73.66,7.87 0 top
U$37  78.74,7.87 0 top
U$38  83.82,7.87 0 top
U$39  88.9,7.87 0 top
U$40  93.98,7.87 0 top
U$41  22.86,7.87 0 top
U$42  27.94,7.87 0 top
U$43  33.02,7.87 0 top
U$44  38.1,7.87 0 top
U$45  43.18,7.87 0 top
U$46  48.26,7.87 0 top
U$47  95.5,54.61 270 top
U$48  10.79,70.74 270 top
U$49  62.7,71.63 180 top
U$50  52.7,71.63 180 top
U$52  24.64,48.77 180 top
U$53  7.62,7.87 0 top

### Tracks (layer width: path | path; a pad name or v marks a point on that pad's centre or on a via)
12V_EN  (via drill 0.6)
  Top 0.406: U$3.27 66.11,50.35 v66.93,49.53 | R57.2 50.19,56.64 v51.18,56.64
  Bottom 0.406: v66.93,49.53 66.04,49.53 58.93,56.64 v51.18,56.64
+5V  (via drill 0.6)
  Top 0.406: v69.6,57.02 69.6,56.01 70.38,55.23 U$3.4 73.51,55.23 76.83,58.55 | v61.21,56.9 58.8,56.9 53.98,52.07 U$7.1 53.98,47.62 53.98,46.35 | v61.21,56.9 61.27,56.83 | 76.83,58.55 SN65.P$3 | U$3.19 61.28,56.83 v61.21,56.9 | 53.98,46.35 45.21,46.35 42.04,49.53 32.38,49.53 29.21,52.7 26.67,52.7 v25.65,53.72 | 53.98,46.35 64.77,46.35 | 64.77,46.35 64.77,47.88 U$14.1 | C16.1 67.18,46.35 64.77,46.35 | 76.83,58.55 v80.52,58.55 R63.1 | IC2.2 19.56,65.86 v19.56,61.59 | v94.36,54.86 97.41,51.82 U$47.8 97.41,48.26 95.76,46.61 C21.1 95,44.7 90.81,40.51 PDS1-S5-S5.2
  Bottom 0.406: v69.6,57.02 61.34,57.02 v61.21,56.9 | v80.52,58.55 81.79,59.82 87.5,59.82 89.41,59.82 v94.36,54.86 | v25.65,53.72 19.56,59.82 v19.56,61.59
+12V
  Top 0.61: T1.E 56.64,62.85 56.64,65.79 56.64,66.29 52.7,70.23 52.7,72.26 51.44,73.53 22.22,73.53 15.9,67.21 IC2.1 14.91,65.53 C7.1 6.73,65.53 6.22,65.02 4.95,63.75 4.95,61.98 4.95,59.18 SPBW06G-12.6
B+
  Top 0.61: U$53.P$1 U$8.P$1 5.08,27.76 F3.1
FD  (via drill 0.6)
  Top 0.61: U$52.P$4 20.27,47.62 21.59,47.62 22.86,48.9 22.86,50.8 21.34,52.32 16.26,52.32 v15.24,53.34 | U$52.P$4 20.32,47.32 | U$52.P$4 20.14,47.06 13.08,40.01 F3.2
  Bottom 0.61: U$48.A2 U$48.A 15.15,72.99 16.51,71.75 16.51,67.31 15.24,66.04 v15.24,53.34
FDS
  Top 0.254: U$8.P$2 7.62,28.96 13.9,35.23 19.05,35.23 | 19.05,35.23 U$5.1 | 19.05,35.23 C3.1
FS
  Top 0.61: U$18.P$2 10.43,25.5 R2.1 9.88,25.22 | U$18.P$2 10.43,22.88 | U$18.P$2 8.89,21.4 8.89,19.68 8.89,11.05 12.06,7.87 U$32.P$1
GND  (via drill 0.6)
  Top 0.254: C5.2 65.19,65.87 v66.04,65.02 66.89,64.17 C4.2
  Top 0.305: U$3.20 64.24,56.03 v64.39,55.88
  Top 0.406: PROG1.1 86.49,49.02 C2.1 87.63,48.01 88.01,47.62 89.53,47.62 89.92,47.24 R14.2 91.79,46.2 C21.2 | U$3.5 72.79,56.03 v73.79,57.02 | U$7.2 52.7,47.88 52.32,47.5 45.47,47.5 45.09,47.88 U$7.8 v45.09,50.67 | U$52.P$2 28.45,50.67 v26.92,50.67 | U$14.2 63.5,47.88 63.12,47.5 56.26,47.5 55.88,47.88 U$14.8 v55.88,50.67 55.88,51.31 C1.1 | C16.2 v72.26,46.99 | C20.2 v82.8,58.55 | C15.2 C11.2 88.65,59.44 88.27,59.05 88.27,53.34 88.65,52.96 C12.2 90.3,52.96 91.44,52.96 v92.71,51.69 93.6,50.8 U$47.5 | v46.48,60.45 46.99,59.94 R51.1 | IC2.4 v17.4,61.59 | v34.67,62.1 33.81,62.97 R53.1
  Top 0.61: SN65.P$2 v75.56,61.98 | R14.2 89.66,45.97 89.66,44.2 89.66,35.69 88.27,34.29 PDS1-S5-S5.1 | T2.E 49.78,61.45 v49.78,60.58 | IC2.4 16.26,62.73 C7.2 8.76,62.73 SPBW06G-12.7
  Bottom 0.406: v26.92,50.67 17.4,60.2 v17.4,61.59 | v46.48,60.45 44.83,62.1 v34.67,62.1
  Bottom 0.61: v26.92,50.67 v45.09,50.67
  pour Bottom: 44.45,45.72 44.45,66.55 53.34,75.44 82.55,75.56 82.55,59.05 94.61,59.05 94.61,46.35
GND2  (via drill 0.6)
  Top 0.254: 78.11,40.01 81.15,40.01 C18.2 | 76.78,40.01 U$1.26 | v77.6,40.01 76.78,40.01 | v77.6,40.01 78.11,40.01 | U$1.27 76.28,40.01 76.78,40.01 | U$14.15 63.5,40.89 63.75,41.15 65.41,41.15 65.66,40.89 65.79,40.77 66.67,39.88 68.96,39.88 69.78,40.69 U$1.40 U$1.39 U$1.38 U$1.37 71.28,40.54 v71.25,40.51 | v77.6,40.01 78.11,40.01 | v55.88,41.91 U$14.9 | C19.1 62.23,34.42 v63.5,33.15 64.77,34.42 C13.2
  Top 0.406: 81.15,40.01 83.31,40.01 C14.2
  Top 0.61: R39.1 91.69,12.69 | C10.2 SPBW06G-12.1
  Top 1.27: 91.69,12.69 v92.71,12.7
  Top 1.778: R39.1 90.17,11.68 U$40.P$1
  Bottom 0.61: v55.88,41.91 55.88,43.18 54.61,44.45 6.99,44.45 SPBW06G-12.1
  pour Bottom: 55.88,43.18 93.34,43.18 93.34,11.18 55.88,11.18
GND3  (via drill 0.6)
  Top 0.254: 24.44,40.01 C3.2 C8.2 | 24.44,40.01 U$5.40 | 24.44,40.01 24.94,40.01 | 24.94,40.01 U$5.39 | 24.94,40.01 25.44,40.01 | 25.44,40.01 U$5.38 | 25.44,40.01 25.94,40.01 | 25.94,40.01 U$5.37 | 25.94,40.01 v26.04,40.01 | U$5.27 30.94,40.13 v31.24,40.13 | v31.24,40.13 31.44,40.13 U$5.26 | C6.2 35.82,40.13 v31.24,40.13
  Top 0.61: R7.1 53.61,25.23 U$9.P$2 52.07,22.94 | v44.96,41.91 45.09,41.91 U$7.9 | v52.58,41.91 52.7,41.91 U$7.15 52.7,37.59 C9.1 | R50.1 49.27,12.69 v50.8,14.22 50.8,21.84 51.9,22.94 52.07,22.94 | U$6.P$1 50.8,24.21 52.07,22.94
  Top 1.778: R50.1 47.5,12.69 52.32,7.87 U$31.P$1
  pour Bottom: 7.37,11.18 53.09,11.18 53.34,42.55 17.78,42.55 7.62,33.02
N$1
  Top 1.27: D1.C 18.27,54.61 U$26.6 22.86,54.61 24.77,56.52 24.77,59.05 27.3,61.59 F1.1
N$2
  Top 0.254: U$1.10 72.28,36.56 72.26,36.58 71.28,36.58 | 71.28,36.58 U$1.8 | 70.28,36.58 U$1.6 | 70.28,36.58 71.28,36.58 | 69.28,36.58 U$1.4 | 69.28,36.58 70.28,36.58 | 69.28,36.58 68.28,36.58 U$1.2 68.28,34.37 65.66,31.75 55.63,31.75 53.34,29.46 R7.2
N$3
  Top 0.406: U$47.2 96.14,60.96 97.28,62.1 R60.1 97.28,63.88 96.9,64.26 95.5,64.26 95.12,64.64 C22.1
N$4
  Top 0.254: U$5.42 23.44,42.99 25.15,44.7 37.34,44.7 39.88,42.16 39.88,38.61 41.4,37.08 48.01,37.08 50.16,39.24 U$7.13
N$5
  Top 0.254: U$5.41 23.94,42.73 25.4,44.2 37.08,44.2 39.37,41.91 39.37,38.35 41.15,36.58 48.77,36.58 51.44,39.24 U$7.14
N$6
  Top 0.254: U$5.43 22.94,43.26 24.89,45.21 37.59,45.21 40.39,42.42 40.39,41.27 | 40.39,41.27 40.39,38.86 41.66,37.59 45.97,37.59 47.62,39.24 U$7.11 | R1.2 41.81,41.27 40.39,41.27
N$7
  Top 0.254: U$14.13 60.96,40.89 62.23,42.16 65.91,42.16 66.67,41.4 67.06,41.02 67.69,41.02 68.58,41.02 68.78,41.22 U$1.42
N$8
  Top 0.254: U$5.44 22.44,43.52 24.64,45.72 37.85,45.72 40.64,42.93 46.74,42.93 48.9,40.77 U$7.12
N$9  (via drill 0.6)
  Top 0.254: 27.94,39.62 26.92,38.61 17.4,38.61 16.51,37.72 C8.1 | 27.94,39.62 27.94,40.64 | 27.94,40.64 U$5.33 | 28.44,40.64 U$5.32 | 27.94,40.64 28.44,40.64 | U$5.31 28.94,40.64 28.44,40.64 | 27.94,39.62 30.73,36.83 34.04,36.83 34.04,35.05 v36.32,35.05 | v40.89,35.05 51.43,35.05 C9.2 52.71,34.8 53.09,34.8 53.98,35.69 U$7.16 53.98,42.29 52.58,43.69 42.67,43.69 R1.1
  Bottom 0.254: v36.32,35.05 v40.89,35.05
N$10
  Top 0.254: U$1.23 84.25,42.11 84.96,41.4 84.96,31.24 84.96,30.61 86.36,29.21 R26.2
N$11
  Top 0.254: U$1.41 69.28,40.95 68.71,40.39 66.93,40.39 66.17,41.15 65.66,41.66 62.99,41.66 62.23,40.89 U$14.14
N$12
  Top 0.254: 88.88,28.35 R27.2 88.9,29.21 88.52,29.59 86.74,29.59 85.47,30.86 85.47,32.64 85.47,33.27 85.47,41.66 83.95,43.18 77.85,43.18 77.78,43.1 U$1.24
N$13
  Top 0.254: U$1.25 77.28,43.37 77.6,43.69 84.2,43.69 85.98,41.91 85.98,35.31 85.98,34.67 85.98,31.11 87,30.1 90.55,30.1 91.44,29.21 R28.2 91.69,28.6
N$14
  Top 0.254: U$5.30 29.44,40.16 31.75,37.85 35.3,37.85 C6.1
N$15
  Top 0.254: U$1.43 68.28,42.98 68.07,43.18 60.71,43.18 58.42,40.89 U$14.11
  Top 0.406: R52.2 58.42,38.89 U$14.11
N$16
  Top 0.254: U$1.44 67.78,42.67 61.47,42.67 59.69,40.89 U$14.12
N$17
  Top 0.254: U$5.23 37.01,41.98 37.85,41.15 37.85,34.8 43.18,29.46 R40.2
N$18
  Top 0.254: U$5.24 32.44,43.1 32.51,43.18 36.58,43.18 38.35,41.4 38.35,35.05 43.43,29.97 45.21,29.97 45.72,29.46 R41.2
N$19
  Top 0.254: C2.2 87.51,45.47 75.95,45.47 74.93,46.48 PROG1.5 71.23,51.33 U$3.32
  Top 0.305: U$3.32 U$3.31
N$20
  Top 1.27: U$2.P$2 27.81,71.63 22.23,66.04 F1.2
N$21
  Top 0.254: U$5.25 31.94,43.37 32.26,43.69 36.83,43.69 38.86,41.66 38.86,35.31 43.69,30.48 47.24,30.48 48.26,29.46 R42.2
N$22
  Top 0.254: U$5.12 27.94,33.78 27.18,33.02 17.53,33.02 15.24,30.73 R4.2
N$23
  Top 0.254: U$1.12 73.28,34.03 73.03,33.78 69.22,33.78 66.17,30.73 59.69,30.73 58.42,29.46 R9.2
N$24
  Top 0.254: U$1.14 74.28,33.51 73.53,32.77 69.72,32.77 66.67,29.72 63.75,29.72 63.5,29.46 R11.2
N$25
  Top 0.254: C18.1 81.15,37.47 75.56,37.47 74.28,38.76 74.28,39.37 | 74.28,40.77 U$1.31 | 73.78,40.77 U$1.32 | 74.28,40.77 73.78,40.77 | U$1.33 73.28,40.77 73.78,40.77 | 74.28,39.37 74.28,40.77 | 64.77,39.37 U$14.16 | 64.77,39.37 73.66,39.37 74.28,39.37 | 64.77,39.37 64.77,39.24 64.39,38.86 62.61,38.86 62.23,38.48 C19.2 59.69,35.05 R52.1
N$26
  Top 0.254: U$1.16 75.28,32.98 74.04,31.75 70.23,31.75 68.58,30.1 R18.2
N$27
  Top 0.254: R21.2 73.66,29.46 76.28,32.08 U$1.18
N$28
  Top 0.254: U$1.20 77.28,31.31 78.74,29.84 R23.2
N$29
  Top 0.254: U$1.22 78.28,31.83 79.88,30.23 82.8,30.23 83.82,29.21 R25.2
N$30
  Top 0.254: U$5.14 28.94,33.25 27.69,32 21.59,32 20.32,30.73 R6.2
N$31
  Top 0.254: U$5.16 29.94,32.73 28.19,30.99 25.65,30.99 25.4,30.73 R15.2
N$32
  Top 0.254: U$3.2 77.76,53.63 77.98,53.85 79.5,53.85 80.01,53.34 80.01,50.8 80.64,50.16 82.55,50.16 | 82.55,50.16 PROG1.2 | LD1.AX 83.82,51.44 82.55,50.16
N$33
  Top 0.254: U$3.1 77.98,52.83 LD1.AR 78.74,48.9 PROG1.3
N$34
  Top 1.27: F2.2 37.47,68.89 U$28.P$2
N$35
  Top 0.406: C1.2 59.8,55.23 U$3.21
N$36
  Top 0.254: SN65.P$4 78.11,61.85 76.96,62.99 74.42,62.99 73.41,61.98 73.41,58.93 72.23,57.75 U$3.7
N$37
  Top 0.254: U$3.6 72.19,56.83 74.3,58.93 SN65.P$1
N$38
  Top 0.406: SN65.P$7 75.56,66.67 74.42,67.82 59.65,67.82 U$50.P$1
N$39
  Top 0.406: SN65.P$6 76.83,66.67 74.8,68.71 63.76,68.71 U$49.P$2
N$40
  Top 0.406: R61.1 94.85,62.84 C22.2 94.87,62.61 U$47.3
N$41
  Top 0.406: U$29.P$1 81.81,71.63 R55.1
N$42
  Top 0.61: SPBW06G-12.2 6.61,47.88 C10.1 15.5,47.88 D2.C
N$43  (via drill 0.6)
  Top 0.61: U$52.P$3 20.07,50.16 17.01,50.16 D2.A 14.74,50.67 v13.97,51.44
  Bottom 0.61: U$48.B2 U$48.B 13.97,68.23 v13.97,51.44
N$44
  Top 0.61: R62.1 50.2,66.04 U$50.P$2
N$45
  Top 0.254: LD1.C 81.28,52.7 82.55,53.98 84.45,53.98 85.09,53.34 85.09,52.07 86.87,50.29 89.41,50.29 90.17,49.53 R14.1
N$46
  Top 0.254: U$5.18 30.94,30.07 R17.2
N$47
  Top 0.254: U$3.8 72.27,58.55 72.9,59.18 72.9,64.26 SN65.P$8
N$48
  Top 0.254: U$3.10 69.31,61.69 70.1,62.48 71.63,62.48 72.14,62.99 72.14,65.28 71.63,65.79 70.7,65.79 C4.1 70.26,66.22 Q1.3
N$49
  Top 0.254: U$3.11 68.51,61.03 65.79,63.75 63.91,63.75 Q1.1 61.82,63.82 C5.1
N$50
  Top 0.254: U$5.20 31.94,34.1 35.56,30.48 R29.2
N$51
  Top 0.254: U$5.22 32.94,34.63 36.07,31.5 39.88,31.5 40.64,30.73 R31.2
N$52
  Top 0.406: U$47.7 96.14,51.31 90.17,57.28 R54.2
N$53
  Top 1.27: D1.A 18.27,59.69 U$26.4 22.23,59.69 24.77,62.23 24.77,65.41 26.67,67.31 30.48,67.31 35.2,70.77 U$2.P$1
N$54
  Top 0.61: R3.1 12.43,25.5 U$18.P$1
N$55
  Top 0.61: R5.1 17.51,25.5 U$19.P$1
N$56
  Top 0.61: R13.1 22.59,25.5 U$20.P$1
N$57
  Top 0.61: R8.1 55.61,25.23 U$9.P$1
N$58
  Top 0.61: U$10.P$1 60.69,25.23 R10.1
N$59
  Top 0.61: U$11.P$1 65.77,25.23 R12.1
N$60
  Top 0.61: U$17.P$1 91.17,25.23 R28.1
N$61
  Top 0.61: U$12.P$1 70.85,25.23 R19.1
N$62
  Top 0.61: U$13.P$1 75.93,25.23 R22.1
N$63
  Top 0.61: U$15.P$1 81.01,25.23 R24.1
N$64
  Top 0.61: U$16.P$1 86.09,25.23 R26.1
N$65
  Top 0.61: R27.1 89.17,25.23 U$17.P$2 87.63,21.4 87.63,12.95 87.37,12.69 R38.1
  Top 1.778: R38.1 85.09,11.68 U$39.P$1
N$66
  Top 0.254: U$1.30 74.78,39.14 75.18,38.73 83.19,38.73 83.44,38.48 C14.1
N$67
  Top 0.61: R42.1 47.99,25.5 U$25.P$1
N$68
  Top 0.61: R16.1 27.67,25.5 U$21.P$1
N$69
  Top 0.61: R25.1 84.09,25.23 U$16.P$2 82.55,21.4 82.55,12.95 82.29,12.69 R37.1
  Top 1.778: 80.23,12.69 R37.1 80.01,11.68 U$38.P$1
N$70
  Top 0.61: R23.1 79.01,25.23 U$15.P$2 77.47,21.4 77.47,12.95 77.21,12.69 R36.1
  Top 1.778: R36.1 74.93,11.68 U$37.P$1
N$71
  Top 0.61: R38.2 U$16.P$3
N$72
  Top 0.61: R39.2 U$17.P$3
N$73
  Top 0.61: R37.2 U$15.P$3
N$74
  Top 0.61: R21.1 73.93,25.23 U$13.P$2 72.39,21.4 72.39,12.95 72.13,12.69 R35.1
  Top 1.778: R35.1 69.85,11.68 U$36.P$1
N$75
  Top 0.61: R36.2 U$13.P$3
N$76
  Top 0.61: R18.1 68.85,25.23 U$12.P$2 67.31,21.4 67.31,12.95 67.05,12.69 R34.1
  Top 1.778: R34.1 64.77,11.68 U$35.P$1
N$77
  Top 0.61: R35.2 U$12.P$3
N$78
  Top 0.61: R11.1 63.77,25.23 U$11.P$2 62.23,21.4 62.23,12.95 61.97,12.69 R33.1
  Top 1.778: R33.1 59.69,11.68 U$34.P$1
N$79
  Top 0.61: R32.1 56.89,12.69 57.15,12.95 57.15,21.4 U$10.P$2 58.69,25.23 R9.1
  Top 1.778: R32.1 54.61,11.68 U$33.P$1
N$80
  Top 0.61: R33.2 U$10.P$3
N$81
  Top 0.61: R34.2 U$11.P$3
N$82
  Top 0.61: R32.2 U$9.P$3
N$83
  Top 0.254: U$1.21 77.78,31.57 79.63,29.72 80.77,29.72 81.28,29.21 R24.2
N$84
  Top 0.254: U$1.19 76.78,29.04 R22.2
N$85
  Top 0.61: R20.1 32.75,25.5 U$22.P$1
N$86
  Top 0.61: R30.1 37.83,25.5 U$23.P$1
N$87
  Top 0.61: R40.1 42.91,25.5 U$24.P$1
N$88
  Top 0.61: R41.1 45.99,25.5 U$25.P$2 44.45,21.4 44.45,12.95 44.19,12.69 R49.1
  Top 1.778: R49.1 42.42,12.69 47.24,7.87 U$46.P$1
N$89
  Top 0.254: U$1.11 72.78,34.55 72.77,34.54 72.77,34.29 68.96,34.29 65.91,31.24 57.66,31.24 55.88,29.46 R8.2
N$90
  Top 0.254: U$1.13 73.78,33.77 73.28,33.27 69.47,33.27 66.42,30.23 61.72,30.23 60.96,29.46 R10.2
N$91
  Top 0.254: U$1.15 74.78,33.25 73.79,32.26 69.98,32.26 66.04,28.32 R12.2
N$92
  Top 0.61: R31.1 40.91,25.5 U$24.P$2 39.37,21.4 39.37,12.95 39.11,12.69 R48.1
  Top 1.778: R48.1 37.34,12.69 42.16,7.87 U$45.P$1
N$93
  Top 0.254: U$1.17 75.78,32.72 74.3,31.24 72.9,31.24 71.12,29.46 R19.2
N$94
  Top 0.61: R29.1 35.83,25.5 U$23.P$2 34.29,21.4 34.29,12.95 34.03,12.69 R47.1
  Top 1.778: R47.1 32.26,12.69 37.08,7.87 U$44.P$1
N$95
  Top 0.61: R49.2 U$24.P$3
N$96
  Top 0.61: R50.2 U$25.P$3
N$97
  Top 0.61: R48.2 U$23.P$3
N$98
  Top 0.61: R17.1 30.75,25.5 U$22.P$2 29.21,21.4 29.21,12.95 28.95,12.69 R46.1
  Top 1.778: R46.1 27.18,12.69 32,7.87 U$43.P$1
N$99
  Top 0.61: R47.2 U$22.P$3
N$100
  Top 0.61: R15.1 25.67,25.5 U$21.P$2 24.13,21.4 24.13,12.95 23.87,12.69 R45.1
  Top 1.778: R45.1 22.1,12.69 26.92,7.87 U$42.P$1
N$101
  Top 0.61: R46.2 U$21.P$3
N$102
  Top 0.61: R6.1 20.59,25.5 U$20.P$2 19.05,21.4 19.05,12.95 18.79,12.69 R44.1
  Top 1.778: R44.1 17.02,12.69 21.84,7.87 U$41.P$1
N$103
  Top 0.61: R4.1 15.51,25.5 U$19.P$2 13.97,21.4 13.97,12.95 13.71,12.69 R43.1
  Top 1.778: R43.1 11.94,12.69 16.76,7.87 U$30.P$1
N$104
  Top 0.61: R44.2 U$19.P$3
N$105
  Top 0.61: R45.2 U$20.P$3
N$106
  Top 0.61: R43.2 U$18.P$3
N$107
  Top 0.254: U$5.11 27.44,34.04 26.92,33.53 15.49,33.53 12.7,30.73 R3.2
N$108
  Top 0.254: U$5.13 28.44,33.52 27.43,32.51 19.56,32.51 17.78,30.73 R5.2
N$109
  Top 0.254: U$5.15 29.44,32.99 27.94,31.5 23.62,31.5 22.86,30.73 R13.2
N$110
  Top 0.254: U$5.17 30.44,32.47 27.94,29.97 R16.2
N$111
  Top 0.254: U$5.19 31.44,33.84 33.02,32.26 R20.2
N$112
  Top 0.254: U$5.21 32.44,34.37 35.81,30.99 37.85,30.99 38.1,30.73 R30.2
N$113
  Top 0.254: R2.2 10.16,30.73 13.46,34.04 22.94,34.04 | 25.94,34.04 U$5.8 | 24.94,34.04 U$5.6 | 24.94,34.04 25.94,34.04 | 23.94,34.04 U$5.4 | 23.94,34.04 24.94,34.04 | 22.94,34.04 U$5.2 | 22.94,34.04 23.94,34.04 | U$5.10 26.94,34.3 26.67,34.04 25.94,34.04
N$114
  Top 0.406: U$29.P$3 72.87,69.6 76.05,69.6 R56.1 80.52,65.13 R63.2
N$115
  Top 1.27: F2.1 42.55,61.59 40.01,59.05 40.01,56.52 38.1,54.61 U$27.6 33.51,54.61 D3.C
N$116
  Top 0.406: PDS1-S5-S5.5 95.89,43.56 C17.1 98.93,46.61 98.93,47.88 98.93,58.29 97.41,59.82
  Top 0.61: 97.41,59.82 U$47.1
N$117
  Top 1.27: U$28.P$1 40.01,66.43 40.01,62.23 37.47,59.69 U$27.4 33.51,59.69 D3.A
N$118
  Top 0.254: U$3.14 66.11,60.89 65.28,61.72 58.93,61.72 48.9,51.69 32.77,51.69 29.84,54.61 U$26.1
N$119
  Top 0.254: U$3.13 66.91,60.85 65.53,62.23 58.55,62.23 50.93,54.61 50.42,54.1 45.85,54.1 44.96,54.1 U$27.1
N$120
  Top 0.406: U$26.2 30.96,58.9 R53.2
N$121
  Top 0.406: R51.2 45.57,57.15 U$27.2
N$122
  Top 0.406: T2.B 47.06,61.53 49.28,59.31 R57.1
N$123
  Top 0.61: T2.C 48.7,63.78 R58.2
N$124  (via drill 0.6)
  Top 0.406: v98.93,41.4 98.93,43.18 C17.2
  Top 0.61: PDS1-S5-S5.4 98.93,35.43 v98.93,41.4 | U$47.4 93.6,59.05 v94.87,57.78
  Bottom 0.61: v98.93,41.4 98.93,57.53 98.55,57.78 v94.87,57.78
N$125
  Top 0.61: T1.B 52.83,60.94 R58.1
N$126
  Top 0.61: R62.2 53.55,66.04 T1.C
N$127
  Top 0.406: U$47.6 94.87,51.18 90.93,55.12 R59.2
N$128
  Top 0.406: R64.2 29.21,47.62 U$52.P$1
N$129
  Top 0.406: SHUNT.P$2 86.51,71.63 86.89,71.63 R61.2
N$130
  Top 0.406: R60.2 97.28,66.29 96.39,67.18 94.65,67.18 92.58,67.18 90.2,69.56 SHUNT.P$1
NEG  (via drill 0.6)
  Top 0.254: U$3.17 63.14,58.42 65.79,58.42 66.8,57.4 v66.8,54.86 | v77.72,54.74 85.19,54.74 85.57,55.12 R59.1 86.84,52.98 C12.1
  Bottom 0.254: v77.72,54.74 76.58,53.59 70.36,53.59 69.6,52.83 68.71,52.83 66.8,54.74 v66.8,54.86
POS  (via drill 0.6)
  Top 0.254: U$3.18 64.04,57.63 v65.79,55.88 | 86.84,57.15 R54.1 85.98,57.28 84.58,55.88 v78.74,55.88 | 86.84,59.41 C11.1
  Top 0.406: R54.1 86.84,59.41
  Bottom 0.254: v65.79,55.88 v78.74,55.88
PWR_HOLD
  Top 0.406: R64.1 42.67,47.62 44.96,45.34 54.61,45.34 68.83,45.34 69.22,45.72 69.22,48.9 67.71,50.4 U$3.29
SLEEP  (via drill 0.6)
  Top 0.254: U$3.30 68.51,53.02 v69.22,53.72 | v76.2,54.99 78.11,56.9 82.3,56.9 83.57,56.9 85.09,58.42 85.09,60.71 85.98,61.59 C15.1 | 86.86,63.73 R55.2
  Top 0.406: C15.1 86.86,63.73
  Bottom 0.254: v69.22,53.72 69.6,54.1 75.31,54.1 v76.2,54.99
TEMP  (via drill 0.6)
  Top 0.254: U$3.28 66.91,53.32 v68.2,54.61 | v74.8,54.99 77.34,57.53 83.31,57.53 84.45,58.67 84.45,61.34 C20.1
  Top 0.406: C20.1 82.8,65.13 R56.2
  Bottom 0.254: v68.2,54.61 74.42,54.61 v74.8,54.99
V+
  Top 0.254: U$6.P$2 50.8,29.46 53.59,32.26 62.23,32.26 65.41,32.26 67.78,34.63 U$1.1 67.78,36.37 66.67,37.47 64.9,37.47 C13.1
VIA
  Top 0.406: U$3.26 65.31,50.45 65.15,50.29 65.02,50.16 62.61,50.16 62.23,49.78 U$14.3
VIA2  (via drill 0.6)
  Top 0.254: U$7.3 51.44,50.55 59.56,58.67 v60.33,58.67 | U$3.9 70.11,60.46 v71.12,61.21
  Bottom 0.406: v71.12,61.21 62.61,61.21 60.58,58.93 v60.33,58.67
VIB
  Top 0.406: U$3.24 61.84,52.83 60.96,51.94 U$14.4
VIB2
  Top 0.254: U$7.4 50.16,50.29 59.56,59.69 63.25,59.69 64.01,58.93 67.71,58.93 | PROG1.4 77.47,48.26 73.79,51.94 70.99,51.94 70.36,52.58 70.36,54.23 67.71,56.88 67.71,58.93 | 67.71,58.93 U$3.12
VIC
  Top 0.406: U$3.23 61.5,53.63 59.69,51.82 U$14.5
VIC2
  Top 0.254: U$7.5 48.9,49.91 59.31,60.33 64.24,60.33 U$3.16
VOD
  Top 0.406: U$3.22 61.16,54.43 58.42,51.69 U$14.6
VOD2
  Top 0.254: U$7.6 47.62,49.53 59.31,61.21 64.77,61.21 65.31,60.67 U$3.15

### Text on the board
tPlace: GND | ZEVA BMS16 V3.2 (OS Edition)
